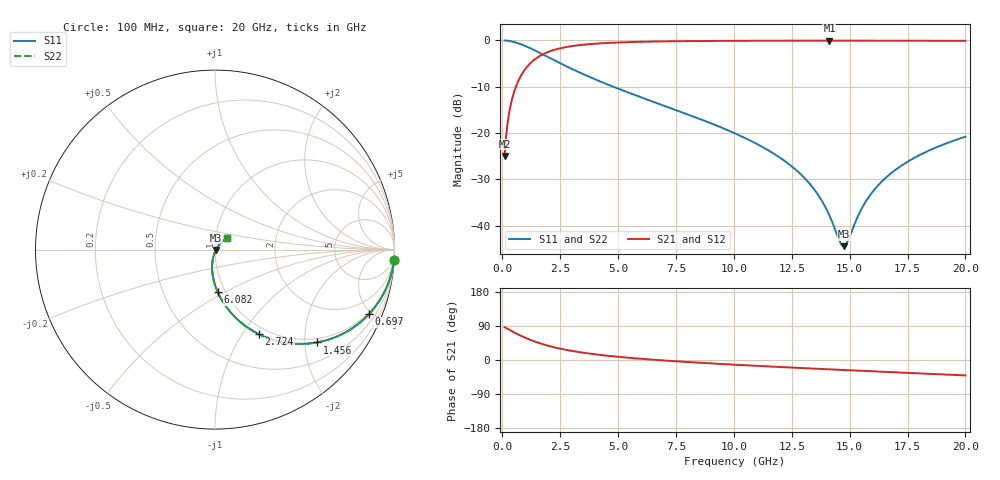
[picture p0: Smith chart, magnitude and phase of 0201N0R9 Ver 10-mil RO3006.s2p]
# GHz S MA R 50
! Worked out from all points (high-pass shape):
!   1601 points, 100 MHz to 20 GHz, reference 50 ohm
!   highest |S21| = -0.05 dB at 14.13 GHz (marker M1); lowest = -25.0 dB at 100 MHz (marker M2)
!   |S21| within 3 dB of the highest: 1.734 GHz to end of sweep
!   lowest |S11| = -44.4 dB at 14.74 GHz (marker M3), VSWR 1.01, Z = 50.5 - j0.281 ohm
!   |S11| at or under -10 dB: 4.791 GHz to end of sweep
!   |S22| runs from -44.4 to 0.0 dB; largest |S21 - S12| = 0
!   S11 on the Smith chart (normalised r, x): 100 MHz: 1, -33; 697 MHz: 0.90, -4.79; 1.456 GHz: 0.90, -2.28; 2.724 GHz: 0.91, -1.19; 6.082 GHz: 0.92, -0.46; 20 GHz: 1.13, +0.15
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0.1  0.9984 -3.4  0.05649 86.6  0.05649 86.6  0.9984 -3.4
0.2616875  0.9892 -8.9  0.1465 81.1  0.1465 81.1  0.9892 -8.9
0.3611875  0.9796 -12.2  0.2003 77.8  0.2003 77.8  0.9796 -12.2
0.697  0.9297 -22.8  0.3674 67.1  0.3674 67.1  0.9297 -22.8
1.032812  0.8618 -32.3  0.5058 57.6  0.5058 57.6  0.8618 -32.3
1.455688  0.7683 -42.3  0.6382 47.6  0.6382 47.6  0.7683 -42.3
2.065125  0.6425 -53.6  0.7638 36.2  0.7638 36.2  0.6425 -53.6
2.724312  0.5314 -62.5  0.8442 27.2  0.8442 27.2  0.5314 -62.5
3.420812  0.4404 -69.7  0.8945 19.9  0.8945 19.9  0.4404 -69.7
6.082438  0.2385 -86.2  0.9669 2.8  0.9669 2.8  0.2385 -86.2
6.741625  0.2076 -89.0  0.9737 -0.2  0.9737 -0.2  0.2076 -89.0
10.05  0.09909 -99.5  0.9898 -12.4  0.9898 -12.4  0.09909 -99.5
12.04  0.05315 -102.7  0.9928 -18.6  0.9928 -18.6  0.05315 -102.7
13.37081  0.02652 -100.0  0.9936 -22.5  0.9936 -22.5  0.02652 -100.0
14.1295  0.01284 -87.4  0.9937 -24.7  0.9937 -24.7  0.01284 -87.4
14.56481  0.006829 -55.1  0.9937 -25.9  0.9937 -25.9  0.006829 -55.1
14.73894  0.005997 -27.7  0.9936 -26.4  0.9936 -26.4  0.005997 -27.7
14.90062  0.00665 -1.8  0.9936 -26.8  0.9936 -26.8  0.00665 -1.8
15.73394  0.0188 41.7  0.9933 -29.1  0.9933 -29.1  0.0188 41.7
16.69162  0.03511 47.8  0.9926 -31.8  0.9926 -31.8  0.03511 47.8
18.09706  0.05902 48.0  0.9912 -35.6  0.9912 -35.6  0.05902 48.0
20  0.09121 44.9  0.9884 -40.7  0.9884 -40.7  0.09121 44.9
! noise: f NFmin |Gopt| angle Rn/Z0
0.1  0.001024  0.9629  1.014  0.006227
2.301  0.005367  0.8269  4.963  0.006508
4.515  0.008288  0.7848  8.796  0.007868
6.729  0.01081  0.7581  12.65  0.008935
8.943  0.01311  0.7387  16.5  0.009843
11.14  0.01527  0.7239  20.29  0.01064
13.36  0.01735  0.7121  24.06  0.01138
15.57  0.01937  0.7028  27.79  0.01206
17.79  0.02135  0.6954  31.47  0.0127
20  0.0233  0.6895  35.09  0.01332
